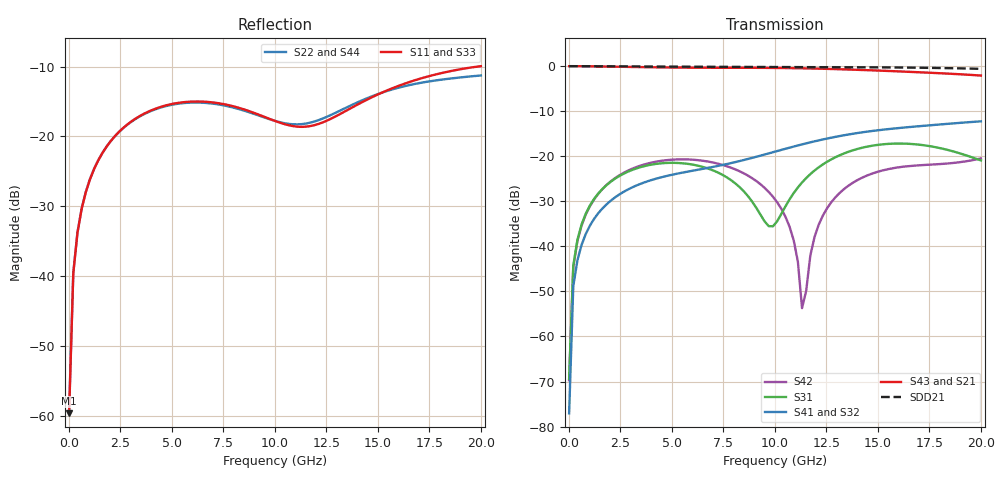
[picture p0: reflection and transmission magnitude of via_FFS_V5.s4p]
! Touchstone file written by Full-Wave Solver - Via VX.2.8
! 2024/08/11, 13:29:59
! HyperLynx Advanced Solvers
! Directory: D:/SERDES_Labs/AA_Example/via_FFS_V5//via_FFS_V5//DUT/
! Project: via_FFS_V5  Simulation: DUT
! User: Terry
! Computer: W10ProDesk
! Single-ended  S-parameters
! HL_PORTMAP 1.0
! PORT 1 +(PIN ENTRY.1, S1, S) NAME:S1||ENTRY.1||GND
! PORT 2 +(PIN EXIT.1, S1, S) NAME:S1||EXIT.1||GND
! PORT 3 +(PIN ENTRY.2, S2, S) NAME:S2||ENTRY.2||GND
! PORT 4 +(PIN EXIT.2, S2, S) NAME:S2||EXIT.2||GND
! CONNECT 1, 2;
! CONNECT 3, 4;
! END_HL_PORTMAP
# HZ S RI R 50
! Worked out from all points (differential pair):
!   100 points, 10 MHz to 20 GHz, reference 50 ohm
!   strongest paths, dB at 10 MHz, 5.058 GHz, 10.11 GHz, 15.15 GHz, 20 GHz:
!     S43: 0.0, -0.3, -0.4, -1.0, -2.1
!     S21: 0.0, -0.3, -0.4, -1.0, -2.1
!     S41: -77.1, -24.1, -18.9, -14.2, -12.3
!     S32: -76.2, -24.1, -18.9, -14.1, -12.3
!     S31: -69.4, -21.5, -34.5, -17.4, -20.9
!     S42: -69.7, -20.7, -30.2, -23.2, -20.5
!   taken as a pair (ports 3,1 in; 4,2 out), SDD21 dB: 0.0, -0.1, -0.2, -0.3, -0.6
!   lowest |S11| = -59.6 dB at 10 MHz (marker M1), VSWR 1.00, Z = 50.1 + j0.0557 ohm
!   |S11| at or under -10 dB: start of sweep to 19.87 GHz
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1e7  0.000886 0.000556  0.999 -0.00282  7.77e-05 0.000328  -5.47e-05 -0.000129
     0.999 -0.00282  0.000955 0.000561  -8.44e-05 -0.00013  7.4e-05 0.000318
     7.77e-05 0.000328  -8.44e-05 -0.00013  0.000865 0.000485  0.999 -0.00289
     -5.47e-05 -0.000129  7.4e-05 0.000318  0.999 -0.00289  0.000957 0.00049
4.138384e8  0.0038 0.02  0.9913 -0.119  0.00181 0.0117  -0.00117 -0.00693
            0.9913 -0.119  0.00338 0.0203  -0.00121 -0.00694  0.00167 0.0114
            0.00181 0.0117  -0.00121 -0.00694  0.00377 0.02  0.9912 -0.1191
            -0.00117 -0.00693  0.00167 0.0114  0.9912 -0.1191  0.00337 0.0202
2.231111e9  0.07 0.0719  0.793 -0.586  0.0376 0.0419  -0.0262 -0.023
            0.793 -0.586  0.0585 0.0814  -0.0263 -0.0228  0.038 0.0424
            0.0376 0.0419  -0.0263 -0.0228  0.0699 0.0719  0.7928 -0.5862
            -0.0262 -0.023  0.038 0.0424  0.7928 -0.5862  0.0584 0.0813
1.091364e10  -0.113 -0.0349  -0.9463 -0.0722  -0.016 0.0356  0.00817 0.1278
             -0.9463 -0.0722  0.1165 -0.0364  0.00886 0.1273  -0.00457 -0.0107
             -0.016 0.0356  0.00886 0.1273  -0.1125 -0.0354  -0.9465 -0.072
             0.00817 0.1278  -0.00457 -0.0107  -0.9465 -0.072  0.1153 -0.0368
1.131747e10  -0.1171 -0.0016  -0.9449 0.0386  -0.00949 0.0503  0.025 0.133
             -0.9449 0.0386  0.1183 -0.0321  0.0255 0.1324  -0.00169 -0.00118
             -0.00949 0.0503  0.0255 0.1324  -0.1167 -0.00217  -0.9451 0.0388
             0.025 0.133  -0.00169 -0.00118  -0.9451 0.0388  0.1171 -0.0323
1.333667e10  -0.0381 0.1443  -0.7459 0.5392  0.0637 0.0859  0.1273 0.1136
             -0.7459 0.5392  0.1541 -0.0318  0.1274 0.1132  0.0393 0.017
             0.0637 0.0859  0.1274 0.1132  -0.0378 0.1439  -0.746 0.5397
             0.1273 0.1136  0.0393 0.017  -0.746 0.5397  0.1527 -0.0318
2e10  0.2186 -0.231  0.6537 0.4365  -0.00412 -0.0898  0.0155 -0.2434
      0.6537 0.4365  0.0643 -0.2652  0.015 -0.2426  -0.0842 -0.043
      -0.00412 -0.0898  0.015 -0.2426  0.2184 -0.2313  0.6538 0.4365
      0.0155 -0.2434  -0.0842 -0.043  0.6538 0.4365  0.0643 -0.264
